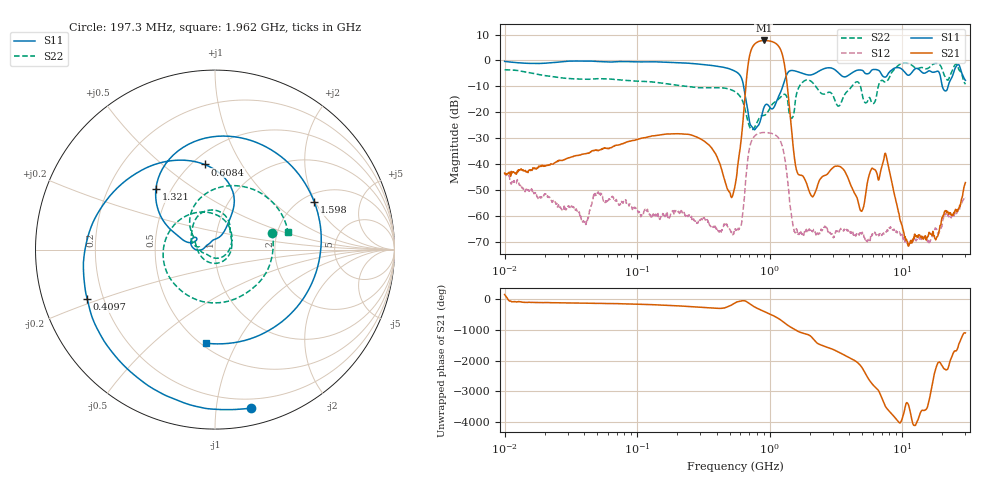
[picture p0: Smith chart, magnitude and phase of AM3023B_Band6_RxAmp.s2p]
# Hz S DB R 50.0
!freq dBS11 angS11 dBS21 angS21 dBS12 angS12 dBS22 angS22
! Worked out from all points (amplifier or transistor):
!   1601 points, 10 MHz to 30 GHz, reference 50 ohm
!   highest |S21| = 7.7 dB at 903.4 MHz (marker M1)
!   |S21| within 3 dB of that: 734.6 MHz to 1.195 GHz (460.7 MHz wide, 47.7 % of centre)
!   unconditionally stable (mu >= 1): start of sweep to end of sweep
!   at 37.85 MHz: K = 1589.31, MAG = -22.6 dB, |S12| = -61.1 dB
!   at 547.7 MHz: K = 142047.30, MAG = -46.2 dB, |S12| = -65.3 dB
!   at 30 GHz: K = 36951.21, MAG = -45.8 dB, |S12| = -52.9 dB
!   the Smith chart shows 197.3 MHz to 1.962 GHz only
!   S11 on the Smith chart (normalised r, x): 197.3 MHz: 0.13, -1.25; 409.7 MHz: 0.14, -0.18; 608.4 MHz: 0.57, +0.71; 1.321 GHz: 0.41, +0.36; 1.598 GHz: 2.32, +1.96; 1.962 GHz: 0.53, -0.76
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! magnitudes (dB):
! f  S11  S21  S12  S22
! 10 MHz  -0.4  -43.5  -43.7  -3.6
! 38.04 MHz  -0.2  -36.3  -61.5  -7.2
! 51.62 MHz  -0.4  -34.7  -51.6  -7.1
! 144.7 MHz  -0.6  -28.9  -60.4  -8.6
! 197.3 MHz  -0.9  -28.3  -58.0  -9.5
! 409.7 MHz  -2.3  -38.4  -65.9  -10.6
! 547.7 MHz  -4.2  -48.5  -65.3  -12.1
! 608.4 MHz  -6.4  -31.0  -63.8  -14.4
! 710.5 MHz  -24.5  2.5  -33.0  -25.9
! 903.4 MHz  -18.3  7.7  -27.8  -21.2
! 1.321 GHz  -6.5  -4.8  -40.1  -13.3
! 1.468 GHz  -3.9  -27.7  -60.7  -22.3
! 1.598 GHz  -4.2  -42.5  -65.2  -12.8
! 1.962 GHz  -5.6  -49.7  -65.7  -7.6
! 2.084 GHz  -5.5  -52.5  -65.7  -8.3
! 3.335 GHz  -5.0  -40.9  -66.3  -17.6
! 4.952 GHz  -3.8  -58.2  -67.0  -12.0
! 5.841 GHz  -3.9  -42.1  -68.1  -16.0
! 7.926 GHz  -4.8  -41.6  -64.9  -7.1
! 11.36 GHz  -5.6  -70.8  -69.6  -1.3
! 18.28 GHz  -4.2  -68.1  -65.4  -1.1
! 30 GHz  -7.7  -47.2  -52.9  -9.2
